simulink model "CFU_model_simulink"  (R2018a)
settings: Solver=ode15s  StartTime=0.0  StopTime=25000  RelTol=1e-6
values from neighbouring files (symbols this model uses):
  D_val = [F_in; ppm_in]    [Casadi_model.m]
  gain_float = [0 1]    [OL_CL_PID.m]
  gain_outflow = [0 1]    [OL_CL_PID.m]
  gain_reject = [0 1]    [OL_CL_PID.m]
  t_float = 16000    [OL_CL_PID.m]
  t_in = 20000    [OL_CL_PID.m]
  t_out = 10000    [OL_CL_PID.m]
  t_ppm = 25000    [OL_CL_PID.m]
  t_Psp = 5000    [OL_CL_PID.m]
  t_reject = 15000    [OL_CL_PID.m]
  U_val = x0_IPOPT(36:38)    [Casadi_model.m]
  x0 = x0_IPOPT(1:35)    [Casadi_model.m]    (also in OL_CL_PID.m = x_initial)
undefined symbols (not defined in the file or in its folder): CFU_model_sim
libraries: simulink x3

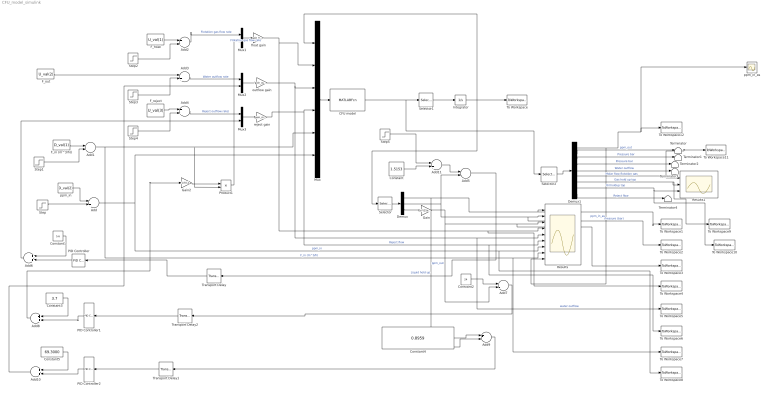
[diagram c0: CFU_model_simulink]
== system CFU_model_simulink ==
  Add{,1..4,6,8,10..11} (9 alike) : Sum
  Add5 : Sum  Inputs=+-
  Add7 : Sum  Inputs=+-
  Add9 : Sum  Inputs=+-
  CFU model : MATLABFcn  MATLABFcn=CFU_model_sim(u(1:35),u(36:38),u(39:40))
  Constant : Constant  Value=1.5153
  Constant1 : Constant  Value=5.6
  Constant2 : Constant  Value=24
  Constant3 : Constant  Value=3.7
  Constant4 : Constant  Value=0.8959
  Constant5 : Constant  Value=69.3000
  Demux : Demux  Outputs=3
  Demux1 : Demux  Outputs=9
  F_float : Constant  Value=U_val(1)
  F_in (m^3/h)) : Constant  Value=D_val(1)
  F_out : Constant  Value=U_val(2)
  F_reject : Constant  Value=U_val(3)
  Gain : Gain  Gain=pi*(25e-6)^3/6 * 1e10*1e6
  Gain2 : Gain  Gain=1/70.2
  Integrator : Integrator  InitialCondition=x0
  Mux : Mux  Inputs=6
  Mux1 : Mux  Inputs=2
  Mux2 : Mux  Inputs=2
  Mux3 : Mux  Inputs=2
  PID Controller : simulink/Continuous/PID Controller  Controller=PI  TimeDomain=Continuous-time  SampleTime=-1  IntegratorMethod=Forward Euler  FilterMethod=Forward Euler  Form=Ideal  UseFilter=on  ControllerParametersSource=internal  P=-55.75  I=1/200  D=0  N=100  InitialConditionSource=internal  InitialConditionForIntegrator=0  InitialConditionForFilter=0  ExternalReset=none  LimitOutput=off  UpperSaturationLimit=inf  LowerSaturationLimit=0  LinearizeAsGain=on  AntiWindupMode=clamping  Kb=1  TrackingMode=off  Kt=1  PParamMin=[]  PParamMax=[]  IParamMin=[]  IParamMax=[]  DParamMin=[]  DParamMax=[]  NParamMin=[]  NParamMax=[]  KbParamMin=[]  KbParamMax=[]  KtParamMin=[]  KtParamMax=[]  POutMin=[]  POutMax=[]  IOutMin=[]  IOutMax=[]  DOutMin=[]  DOutMax=[]  NOutMin=[]  NOutMax=[]  KbOutMin=[]  KbOutMax=[]  KtOutMin=[]  KtOutMax=[]  IntegratorOutMin=[]  IntegratorOutMax=[]  FilterOutMin=[]  FilterOutMax=[]  SumOutMin=[]  SumOutMax=[]  SumI1OutMin=[]  SumI1OutMax=[]  SumI2OutMin=[]  SumI2OutMax=[]  SumI3OutMin=[]  SumI3OutMax=[]  SumDOutMin=[]  SumDOutMax=[]  SaturationOutMin=[]  SaturationOutMax=[]  IntegratorContinuousStateAttributes=''  IntegratorStateMustResolveToSignalObject=off  IntegratorRTWStateStorageClass=Auto  FilterContinuousStateAttributes=''  FilterStateMustResolveToSignalObject=off  FilterRTWStateStorageClass=Auto  DifferentiatorICPrevScaledInput=0  DifferentiatorOutMin=[]  DifferentiatorOutMax=[]  InitialConditionSetting=State (most efficient)  FilterDiffOutCoefMin=[]  FilterDiffOutCoefMax=[]  SumDenOutMin=[]  SumDenOutMax=[]  SumNumOutMin=[]  SumNumOutMax=[]  ReciprocalOutMin=[]  ReciprocalOutMax=[]  DivideOutMin=[]  DivideOutMax=[]  TunerSelectOption=Transfer Function Based (PID Tuner App)
  PID Controller1 : simulink/Continuous/PID Controller  Controller=PI  TimeDomain=Continuous-time  SampleTime=-1  IntegratorMethod=Forward Euler  FilterMethod=Forward Euler  Form=Ideal  UseFilter=on  ControllerParametersSource=internal  P=-0.25  I=1/316  D=0  N=100  InitialConditionSource=internal  InitialConditionForIntegrator=0  InitialConditionForFilter=0  ExternalReset=none  LimitOutput=off  UpperSaturationLimit=inf  LowerSaturationLimit=-inf  LinearizeAsGain=on  AntiWindupMode=none  Kb=1  TrackingMode=off  Kt=1  PParamMin=[]  PParamMax=[]  IParamMin=[]  IParamMax=[]  DParamMin=[]  DParamMax=[]  NParamMin=[]  NParamMax=[]  KbParamMin=[]  KbParamMax=[]  KtParamMin=[]  KtParamMax=[]  POutMin=[]  POutMax=[]  IOutMin=[]  IOutMax=[]  DOutMin=[]  DOutMax=[]  NOutMin=[]  NOutMax=[]  KbOutMin=[]  KbOutMax=[]  KtOutMin=[]  KtOutMax=[]  IntegratorOutMin=[]  IntegratorOutMax=[]  FilterOutMin=[]  FilterOutMax=[]  SumOutMin=[]  SumOutMax=[]  SumI1OutMin=[]  SumI1OutMax=[]  SumI2OutMin=[]  SumI2OutMax=[]  SumI3OutMin=[]  SumI3OutMax=[]  SumDOutMin=[]  SumDOutMax=[]  SaturationOutMin=[]  SaturationOutMax=[]  IntegratorContinuousStateAttributes=''  IntegratorStateMustResolveToSignalObject=off  IntegratorRTWStateStorageClass=Auto  FilterContinuousStateAttributes=''  FilterStateMustResolveToSignalObject=off  FilterRTWStateStorageClass=Auto  DifferentiatorICPrevScaledInput=0  DifferentiatorOutMin=[]  DifferentiatorOutMax=[]  InitialConditionSetting=State (most efficient)  FilterDiffOutCoefMin=[]  FilterDiffOutCoefMax=[]  SumDenOutMin=[]  SumDenOutMax=[]  SumNumOutMin=[]  SumNumOutMax=[]  ReciprocalOutMin=[]  ReciprocalOutMax=[]  DivideOutMin=[]  DivideOutMax=[]  TunerSelectOption=Transfer Function Based (PID Tuner App)
  PID Controller2 : simulink/Continuous/PID Controller  Controller=PI  TimeDomain=Continuous-time  SampleTime=-1  IntegratorMethod=Forward Euler  FilterMethod=Forward Euler  Form=Ideal  UseFilter=on  ControllerParametersSource=internal  P=-318.19  I=1/204  D=0  N=100  InitialConditionSource=internal  InitialConditionForIntegrator=0  InitialConditionForFilter=0  ExternalReset=none  LimitOutput=off  UpperSaturationLimit=inf  LowerSaturationLimit=-inf  LinearizeAsGain=on  AntiWindupMode=none  Kb=1  TrackingMode=off  Kt=1  PParamMin=[]  PParamMax=[]  IParamMin=[]  IParamMax=[]  DParamMin=[]  DParamMax=[]  NParamMin=[]  NParamMax=[]  KbParamMin=[]  KbParamMax=[]  KtParamMin=[]  KtParamMax=[]  POutMin=[]  POutMax=[]  IOutMin=[]  IOutMax=[]  DOutMin=[]  DOutMax=[]  NOutMin=[]  NOutMax=[]  KbOutMin=[]  KbOutMax=[]  KtOutMin=[]  KtOutMax=[]  IntegratorOutMin=[]  IntegratorOutMax=[]  FilterOutMin=[]  FilterOutMax=[]  SumOutMin=[]  SumOutMax=[]  SumI1OutMin=[]  SumI1OutMax=[]  SumI2OutMin=[]  SumI2OutMax=[]  SumI3OutMin=[]  SumI3OutMax=[]  SumDOutMin=[]  SumDOutMax=[]  SaturationOutMin=[]  SaturationOutMax=[]  IntegratorContinuousStateAttributes=''  IntegratorStateMustResolveToSignalObject=off  IntegratorRTWStateStorageClass=Auto  FilterContinuousStateAttributes=''  FilterStateMustResolveToSignalObject=off  FilterRTWStateStorageClass=Auto  DifferentiatorICPrevScaledInput=0  DifferentiatorOutMin=[]  DifferentiatorOutMax=[]  InitialConditionSetting=State (most efficient)  FilterDiffOutCoefMin=[]  FilterDiffOutCoefMax=[]  SumDenOutMin=[]  SumDenOutMax=[]  SumNumOutMin=[]  SumNumOutMax=[]  ReciprocalOutMin=[]  ReciprocalOutMax=[]  DivideOutMin=[]  DivideOutMax=[]  TunerSelectOption=Transfer Function Based (PID Tuner App)
  Product1 : Product
  Results : Scope  NumInputPorts=9
  Results1 : Scope  NumInputPorts=3
  Selector : Selector  InputPortWidth=35  IndexOptions=Index vector (dialog)  Indices=[31 32 33]  OutputSizes=1
  Selector1 : Selector  InputPortWidth=44  IndexOptions=Index vector (dialog)  Indices=[1:35]  OutputSizes=1
  Selector2 : Selector  InputPortWidth=44  IndexOptions=Index vector (dialog)  Indices=[36:44]  OutputSizes=1
  Step : Step  Time=t_ppm  After=10  SampleTime=0
  Step1 : Step  Time=t_in  After=2  SampleTime=0
  Step2 : Step  Time=t_float  After=0.1  SampleTime=0
  Step3 : Step  Time=t_out  After=0.9  SampleTime=0
  Step4 : Step  Time=t_reject  After=0.1  SampleTime=0
  Step5 : Step  Time=t_Psp  After=-0.0453  SampleTime=0
  Terminator{,1..4} (5 alike) : Terminator
  To Workspace : ToWorkspace  VariableName=x_simulink  SampleTime=-1
  To Workspace1 : ToWorkspace  VariableName=liq_hold_up  SampleTime=-1
  To Workspace10 : ToWorkspace  VariableName=oil_hold_up  SampleTime=-1
  To Workspace11 : ToWorkspace  VariableName=mass_flow_flotation  SampleTime=-1
  To Workspace12 : ToWorkspace  VariableName=ppm_in_as  SampleTime=-1
  To Workspace2 : ToWorkspace  VariableName=Pressure  SampleTime=-1
  To Workspace3 : ToWorkspace  VariableName=ppm_out  SampleTime=-1
  To Workspace4 : ToWorkspace  VariableName=F_flotation  SampleTime=-1
  To Workspace5 : ToWorkspace  VariableName=F_out  SampleTime=-1
  To Workspace6 : ToWorkspace  VariableName=F_reject  SampleTime=-1
  To Workspace7 : ToWorkspace  VariableName=F_in  SampleTime=-1
  To Workspace8 : ToWorkspace  VariableName=ppm_in  SampleTime=-1
  To Workspace9 : ToWorkspace  VariableName=gas_hold_up  SampleTime=-1
  Transport Delay : TransportDelay
  Transport Delay1 : TransportDelay  DelayTime=2
  Transport Delay2 : TransportDelay  DelayTime=30
  float gain : Gain  Gain=gain_float  Multiplication=Matrix(K*u)
  outflow gain : Gain  Gain=gain_outflow  Multiplication=Matrix(K*u)
  ppm_in : Constant  Value=D_val(2)
  ppm_in_as : Scope
  reject gain : Gain  Gain=gain_reject  Multiplication=Matrix(K*u)
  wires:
  ppm_in/1 -> Add/1
  Step/1 -> Add/2
  F_in (m^3/h))/1 -> Add1/1
  Step1/1 -> Add1/2
  F_float/1 -> Add2/1
  Step2/1 -> Add2/2
  Step3/1 -> Add3/2
  F_reject/1 -> Add4/1
  Step4/1 -> Add4/2
  Add/1 -> Results/7, To Workspace8/1, Mux/6  "ppm_in"
  Add1/1 -> Results/8, To Workspace7/1, Product1/2, Mux/5  "F_in (m^3/h)"
  outflow gain/1 -> Results/5, To Workspace5/1, Mux/3  "water outflow"
  Add4/1 -> Mux3/1  "Reject outflow rate)"
  Mux/1 -> CFU model/1
  CFU model/1 -> Selector2/1, Selector1/1
  Selector1/1 -> Integrator/1
  Integrator/1 -> To Workspace/1, Selector/1, Mux/1
  Selector/1 -> Demux/1
  Demux/3 -> Gain/1
  Demux/2 -> Add5/2, Results/2, To Workspace2/1  "Pressure (bar)"
  Demux/1 -> Add9/2, To Workspace1/1, Results/1  "Liquid hold up"
  Add2/1 -> Mux1/1  "Flotation gas flow rate"
  Gain/1 -> Results/3, To Workspace3/1, Add7/2  "ppm_out"
  F_out/1 -> Add3/1
  Constant/1 -> Add11/2
  Add5/1 -> Transport Delay/1
  PID Controller/1 -> Add6/2
  Constant1/1 -> Add6/1
  Add6/1 -> Mux3/2
  reject gain/1 -> Results/6, To Workspace6/1, Mux/4  "Reject flow"
  Constant2/1 -> Add7/1
  Add7/1 -> Transport Delay2/1
  Constant3/1 -> Add8/1
  PID Controller1/1 -> Add8/2
  Mux1/1 -> float gain/1  "Flotation gas flow rate"
  Selector2/1 -> Demux1/1
  Demux1/2 -> Terminator/1  "ppm_out"
  Demux1/4 -> Terminator2/1  "Pressure bar"
  Demux1/5 -> Terminator3/1  "Water outflow"
  Demux1/6 -> To Workspace11/1, Results1/1  "Molar flow flotation gas"
  Demux1/7 -> To Workspace9/1, Results1/2  "Gas hold up top"
  Demux1/8 -> To Workspace10/1, Results1/3  "Oil holdup top"
  Demux1/9 -> Terminator4/1  "Reject flow"
  Constant4/1 -> Add9/1
  Add9/1 -> Transport Delay1/1
  Add10/1 -> Mux2/2
  PID Controller2/1 -> Add10/2
  Constant5/1 -> Add10/1
  Add3/1 -> Mux2/1  "Water outflow rate"
  Add11/1 -> Add5/1
  Step5/1 -> Add11/1
  float gain/1 -> Results/4, To Workspace4/1, Mux/2
  Mux2/1 -> outflow gain/1
  Mux3/1 -> reject gain/1
  Transport Delay2/1 -> PID Controller1/1
  Transport Delay1/1 -> PID Controller2/1
  Transport Delay/1 -> PID Controller/1
  Add8/1 -> Gain2/1
  Gain2/1 -> Product1/1
  Product1/1 -> Mux1/2
  Demux1/3 -> Terminator1/1  "Pressure bar"
  Demux1/1 -> Results/9, ppm_in_as/1, To Workspace12/1  "ppm_in_as"
